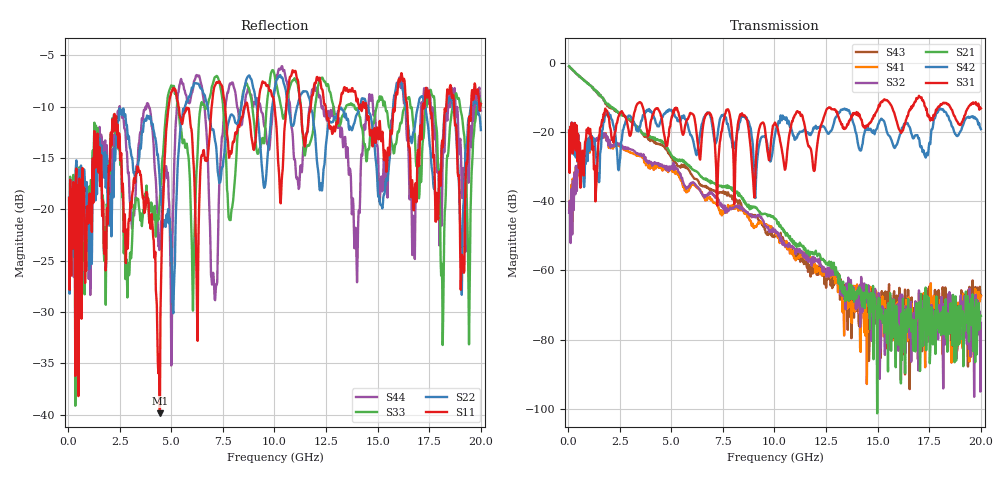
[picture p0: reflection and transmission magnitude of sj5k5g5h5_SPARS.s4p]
! FILE: E:\users\goganessyan\GBX_Backplane\FR408_backplane\1m_INBOUND_TRU\sj5k5g5h5_SPARS.s4p
# MHZ S RI R 50.00
! FREQ  S11  S12  S13  S14
!  S21  S22  S23  S24
!  S31  S32  S33  S34
!  S41  S42  S43  S44
!  REAL  IMAG  REAL  IMAG  REAL  IMAG  REAL  IMAG
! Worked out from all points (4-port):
!   799 points, 50 MHz to 20 GHz, reference 50 ohm
!   strongest paths, dB at 50 MHz, 5.025 GHz, 10.03 GHz, 15.03 GHz, 20 GHz:
!     S31: -19.6, -15.6, -17.3, -13.1, -13.2
!     S42: -19.7, -14.0, -20.6, -17.8, -19.2
!     S21: -1.0, -26.9, -45.1, -69.5, -73.1
!     S32: -43.4, -29.8, -48.2, -76.2, -75.2
!     S41: -42.4, -30.4, -49.1, -70.3, -67.5
!     S43: -1.1, -27.3, -49.7, -74.6, -67.3
!   lowest |S11| = -39.9 dB at 4.45 GHz (marker M1), VSWR 1.02, Z = 51 - j0.224 ohm
!   |S11| at or under -10 dB: start of sweep to 4.874 GHz; 5.353 GHz to 6.958 GHz (1.605 GHz wide, 26.1 % of centre); 14.44 GHz to 15.84 GHz (1.394 GHz wide, 9.21 % of centre)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
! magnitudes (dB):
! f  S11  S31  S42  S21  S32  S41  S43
! 50 MHz  -18.9  -19.6  -19.7  -1.0  -43.4  -42.4  -1.1
! 1.425 GHz  -12.6  -28.7  -34.0  -8.6  -21.7  -21.9  -8.5
! 4.45 GHz  -39.9  -14.4  -17.4  -22.5  -29.5  -30.0  -23.6
! 5.075 GHz  -8.3  -14.5  -14.2  -27.5  -30.3  -31.4  -28.3
! 9 GHz  -14.2  -37.2  -29.5  -41.8  -44.4  -47.8  -44.6
! 14.53 GHz  -11.2  -18.4  -18.4  -66.6  -67.1  -70.6  -70.5
! 20 GHz  -9.7  -13.2  -19.2  -73.1  -75.2  -67.5  -67.3
